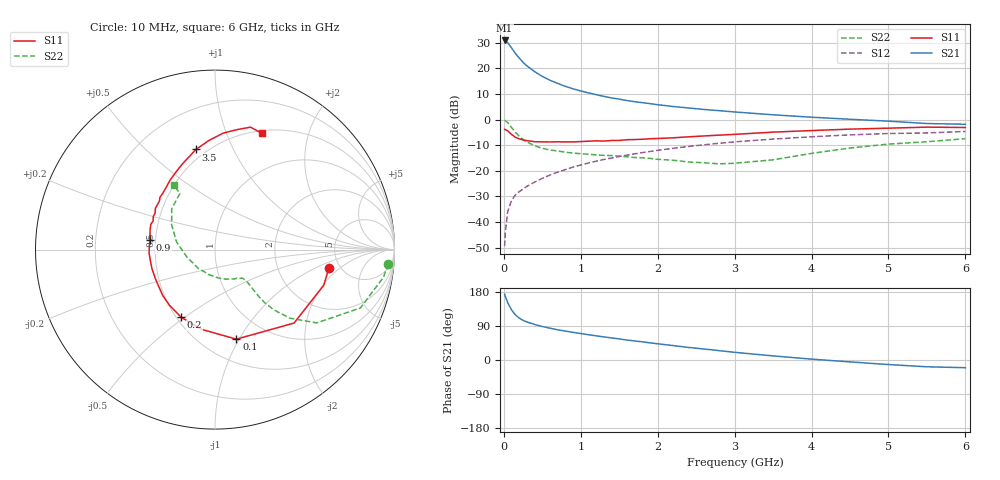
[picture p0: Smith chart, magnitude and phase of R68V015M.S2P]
! SIEMENS Small Signal Semiconductors
! BFR193
! Si NPN RF Bipolar Junction Transistor in SOT23
! VCE = 8 V  IC = 15 mA
! Common Emitter S-Parameters:  May  1996
# GHz  S  MA  R  50
!  f  S11  S21  S12  S22
! GHz  MAG  ANG  MAG  ANG  MAG  ANG  MAG  ANG
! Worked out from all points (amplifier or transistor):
!   36 points, 10 MHz to 6 GHz, reference 50 ohm
!   highest |S21| = 30.8 dB at 10 MHz (marker M1)
!   |S21| within 3 dB of that: start of sweep to 102.4 MHz
!   unconditionally stable (mu >= 1): 666 MHz to 2.071 GHz
!   at 250 MHz: K = 0.74, MSG = 24.7 dB, |S12| = -27.1 dB
!   at 1.4 GHz: K = 1.03, MAG = 10.6 dB, |S12| = -15.0 dB
!   at 6 GHz: K = 0.94, MSG = 1.4 dB, |S12| = -4.7 dB
!   S11 on the Smith chart (normalised r, x): 10 MHz: 4.09, -1.42; 100 MHz: 0.72, -0.97; 200 MHz: 0.53, -0.48; 900 MHz: 0.47, +0.06; 3.5 GHz: 0.44, +0.73; 6 GHz: 0.53, +1.34
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0.01  0.6432 -9.1  34.76 173.7  0.0034 84.7  0.9686 -4.7
0.02  0.6376 -18.2  33.92 167.7  0.0065 82.2  0.9506 -9.4
0.05  0.6012 -42.9  31.41 151.8  0.016 72.1  0.8727 -21.9
0.1  0.513 -76.6  24.91 132.1  0.0265 63.0  0.6981 -35.8
0.15  0.4501 -99.9  19.42 119.2  0.0336 59.3  0.5652 -42.5
0.2  0.421 -116.8  15.78 110.7  0.0392 59.8  0.4712 -45.6
0.25  0.4003 -129.5  13.03 104.7  0.0443 60.1  0.4062 -46.9
0.3  0.3874 -138.9  11.1 100.3  0.0499 61.6  0.3653 -47.0
0.4  0.3701 -153.1  8.583 93.8  0.0603 63.5  0.3088 -46.3
0.5  0.367 -163.1  6.921 88.3  0.0713 64.8  0.2741 -45.5
0.6  0.3654 -170.9  5.828 83.9  0.0829 65.5  0.2551 -45.1
0.7  0.368 -177.3  5.042 79.8  0.0941 65.9  0.2424 -45.2
0.9  0.3663 171.7  3.967 72.9  0.1183 65.5  0.2219 -46.2
1.1  0.378 163.1  3.307 66.7  0.1421 64.9  0.2106 -49.4
1.3  0.3801 155.2  2.827 60.9  0.1665 63.4  0.2001 -52.8
1.6  0.4042 145.2  2.344 52.7  0.2022 60.4  0.1877 -60.6
2.2  0.4398 128.4  1.796 38.1  0.2746 53.5  0.161 -82.0
3  0.5138 110.1  1.403 20.3  0.3668 42.4  0.1404 -130.9
3.5  0.5678 100.8  1.236 10.8  0.4159 34.9  0.1638 -166.5
4.5  0.6499 86.1  1.012 -5.0  0.502 20.7  0.2782 150.3
5.5  0.7105 73.8  0.836 -17.9  0.5481 6.1  0.3689 122.0
6  0.6982 68.0  0.809 -20.3  0.5852 1.9  0.4239 122.5
